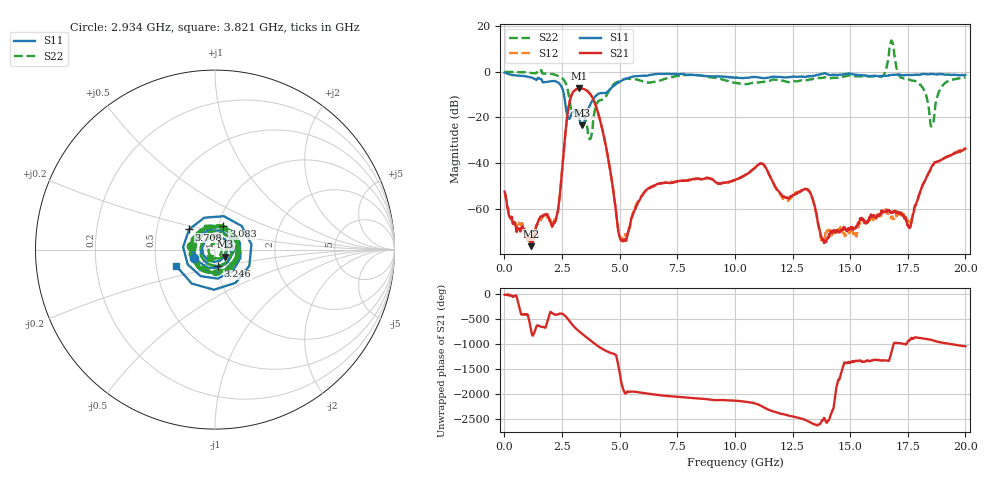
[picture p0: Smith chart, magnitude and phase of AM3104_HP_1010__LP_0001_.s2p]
!Created with skrf (http://scikit-rf.org).
# Hz S RI R 50.0
!freq ReS11 ImS11 ReS21 ImS21 ReS12 ImS12 ReS22 ImS22
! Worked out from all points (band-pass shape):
!   1601 points, 10 MHz to 20 GHz, reference 50 ohm
!   highest |S21| = -7.30 dB at 3.258 GHz (marker M1); lowest = -76.3 dB at 1.172 GHz (marker M2)
!   |S21| within 3 dB of the highest: 2.91 GHz to 3.763 GHz (853.2 MHz wide, 25.6 % of centre)
!   lowest |S11| = -23.4 dB at 3.358 GHz (marker M3), VSWR 1.14, Z = 55.6 - j4.36 ohm
!   |S11| at or under -10 dB: 2.582 GHz to 4.03 GHz (1.448 GHz wide, 43.8 % of centre)
!   |S22| runs from -29.5 to 13.7 dB; largest |S21 - S12| = 0.02
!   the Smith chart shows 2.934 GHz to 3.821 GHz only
!   S11 on the Smith chart (normalised r, x): 2.934 GHz: 0.79, -0.08; 3.083 GHz: 1.06, +0.28; 3.246 GHz: 1.01, -0.19; 3.708 GHz: 0.73, +0.17; 3.821 GHz: 0.63, -0.12
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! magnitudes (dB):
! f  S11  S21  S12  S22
! 10 MHz  -0.4  -52.4  -52.8  0.0
! 1.172 GHz  -2.5  -76.3  -73.3  -0.6
! 2.246 GHz  -4.3  -64.0  -64.1  -1.5
! 2.934 GHz  -18.0  -9.7  -9.8  -17.3
! 3.083 GHz  -17.1  -7.9  -7.9  -17.0
! 3.246 GHz  -20.5  -7.3  -7.4  -17.5
! 3.258 GHz  -20.8  -7.3  -7.4  -17.5
! 3.346 GHz  -23.4  -7.3  -7.4  -18.0
! 3.358 GHz  -23.4  -7.4  -7.4  -18.2
! 3.708 GHz  -14.8  -9.5  -9.5  -29.5
! 3.821 GHz  -12.6  -11.3  -11.3  -25.0
! 5.082 GHz  -3.9  -73.6  -73.0  -3.7
! 6.682 GHz  -0.9  -49.0  -49.1  -4.0
! 10.01 GHz  -2.6  -47.5  -47.4  -4.9
! 11.15 GHz  -2.7  -40.1  -40.3  -4.5
! 13.34 GHz  -2.0  -54.9  -54.6  -3.3
! 13.88 GHz  -0.7  -74.8  -73.1  -2.5
! 16.68 GHz  -1.5  -61.0  -62.1  7.2
! 17.58 GHz  -1.4  -68.4  -66.4  -3.5
! 18.54 GHz  -0.9  -41.5  -41.7  -23.9
! 19 GHz  -1.2  -38.4  -38.2  -6.2
! 20 GHz  -1.4  -33.7  -33.5  -2.5
